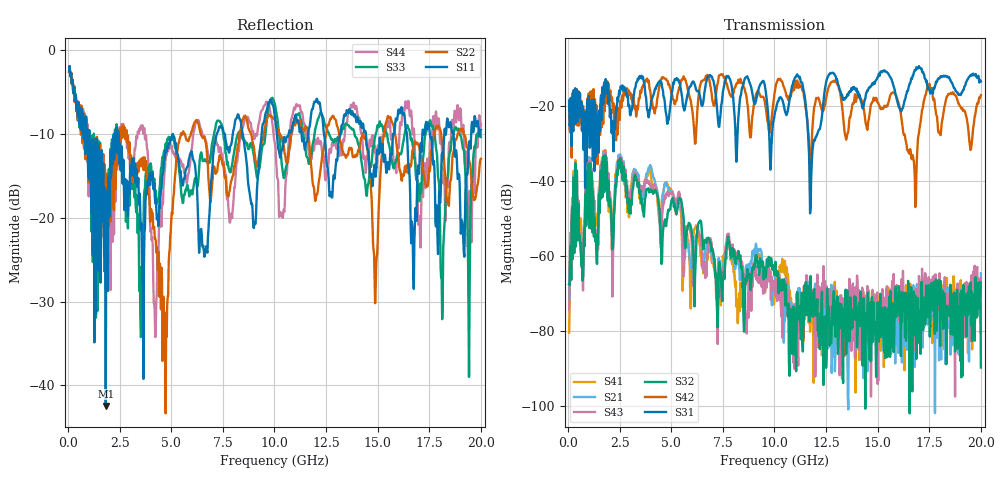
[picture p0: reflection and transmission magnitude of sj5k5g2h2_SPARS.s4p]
! FILE: E:\users\goganessyan\GBX_Backplane\FR408_backplane\1m_OUTBOUND_FEXT\sj5k5g2h2_SPARS.s4p
# MHZ S RI R 50.00
! FREQ  S11  S12  S13  S14
!  S21  S22  S23  S24
!  S31  S32  S33  S34
!  S41  S42  S43  S44
!  REAL  IMAG  REAL  IMAG  REAL  IMAG  REAL  IMAG
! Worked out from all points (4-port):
!   799 points, 50 MHz to 20 GHz, reference 50 ohm
!   strongest paths, dB at 50 MHz, 5.025 GHz, 10.03 GHz, 15.03 GHz, 20 GHz:
!     S31: -18.6, -16.3, -21.7, -12.2, -13.5
!     S42: -19.1, -16.7, -15.9, -19.2, -17.1
!     S32: -67.6, -45.0, -63.4, -75.1, -89.7
!     S43: -74.3, -42.9, -68.6, -75.2, -65.9
!     S21: -65.3, -42.7, -64.9, -93.3, -64.6
!     S41: -80.4, -42.6, -68.1, -75.6, -80.3
!   lowest |S11| = -42.5 dB at 1.825 GHz (marker M1), VSWR 1.02, Z = 50.7 + j0.346 ohm
!   |S11| at or under -10 dB: 2.434 GHz to 5.069 GHz (2.635 GHz wide, 70.2 % of centre); 5.077 GHz to 7.202 GHz (2.125 GHz wide, 34.6 % of centre); 14.43 GHz to 15.75 GHz (1.319 GHz wide, 8.74 % of centre)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
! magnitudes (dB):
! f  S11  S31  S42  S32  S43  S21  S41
! 50 MHz  -2.5  -18.6  -19.1  -67.6  -74.3  -65.3  -80.4
! 1.825 GHz  -42.5  -12.8  -14.2  -42.1  -41.2  -40.9  -42.3
! 8.675 GHz  -13.9  -12.1  -19.0  -63.5  -75.6  -62.4  -67.5
! 11.75 GHz  -8.2  -46.9  -42.2  -65.3  -66.3  -68.8  -75.4
! 12.72 GHz  -16.9  -11.2  -13.8  -83.0  -71.0  -76.8  -70.2
! 16.8 GHz  -20.7  -10.4  -39.4  -81.2  -81.1  -89.6  -69.7
! 20 GHz  -9.5  -13.5  -17.1  -89.7  -65.9  -64.6  -80.3
